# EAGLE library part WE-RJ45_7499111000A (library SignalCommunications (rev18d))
Order Code 7499111000A Design THT xBase-T 10/100/1000 Base-T Ports 1x1 Application Standard Tab Position UP LED (Left-Right) NONE EMI Fingers Yes Details see: http://katalog.we-online.de/en/pbs/WE-LAN_RJ45/7499111000A? Updated by Yingchun Shan 2016-08-29 2016(C) Würth Elektronik
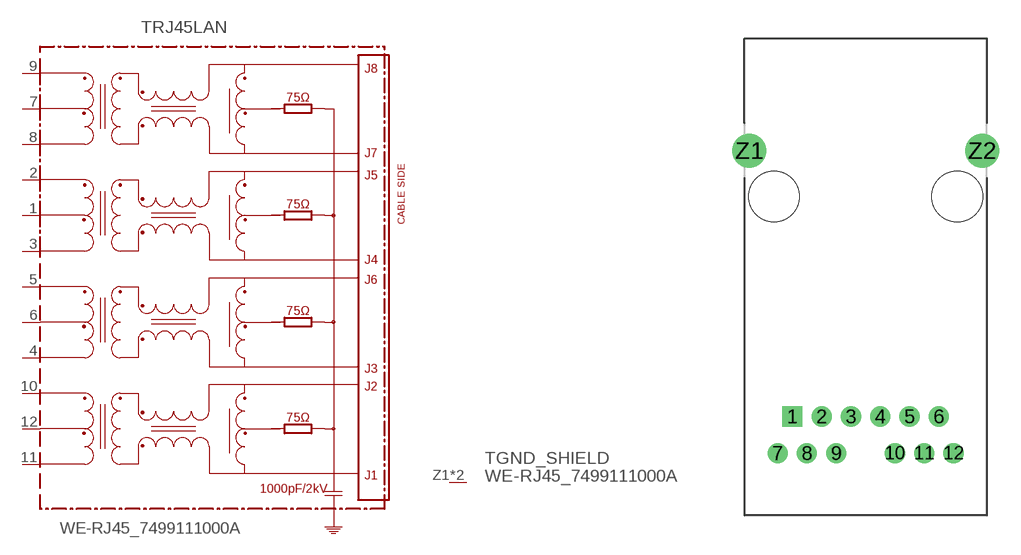
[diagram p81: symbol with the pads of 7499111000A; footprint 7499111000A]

Designator prefix T; gates RJ45LAN=7499111221A/7499111000A GND_SHIELD=GNDPIN

## WE-RJ45_7499111000A (COMPANY-URL: http://www.we-online.de; CREATED-BY: Christin Zierenner; CREATED-DATE: AUG 2012; DATASHEET-URL: http://katalog.we-online.de/kataloge/eisos/media/pdf/7499111000A.pdf; MANUFACTURER: Würth Elektronik eiSos GmbH)  [7499111000A]
1  RJ45LAN:1
2  RJ45LAN:2
3  RJ45LAN:3
4  RJ45LAN:4
5  RJ45LAN:5
6  RJ45LAN:6
7  RJ45LAN:7
8  RJ45LAN:8
9  RJ45LAN:9
10  RJ45LAN:10
11  RJ45LAN:11
12  RJ45LAN:12
Z1  GND_SHIELD:GND  pwr
Z2  GND_SHIELD:GND  pwr

## Footprint 7499111000A (pad centres in mm)
MAX HEIGHT=15.79mm PORTS----1X1 LED --NO
drill 0.89 square: 1 -5.075,-15.24
drill 0.89: 2 -3.045,-15.24; 3 -1.015,-15.24; 4 1.015,-15.24; 5 3.045,-15.24; 6 5.075,-15.24; 7 -6.095,-17.78; 8 -4.065,-17.78; 9 -2.035,-17.78; 10 2.035,-17.78; 11 4.065,-17.78; 12 6.095,-17.78
drill 1.57: Z1 -8.065,3.18; Z2 8.065,3.18
hole 3.5 at 6.35,0
hole 3.5 at -6.35,0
